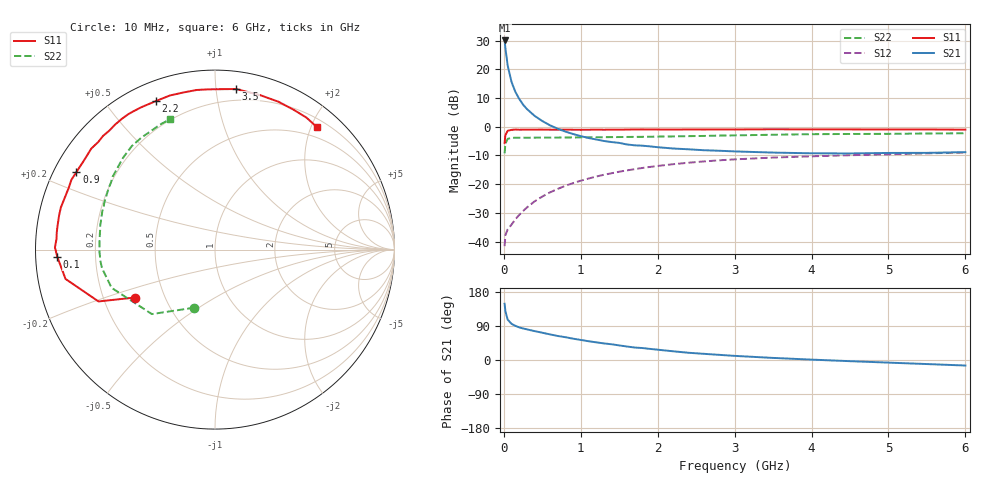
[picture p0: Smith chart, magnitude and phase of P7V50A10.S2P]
! SIEMENS Small Signal Semiconductors
! BFP196
! Si NPN RF Bipolar Junction Transistor in SOT143
! VCE = 0.5 V  IC = 100 mA
! Common Emitter S-Parameters:  May  1996
# GHz  S  MA  R  50
!  f  S11  S21  S12  S22
! GHz  MAG  ANG  MAG  ANG  MAG  ANG  MAG  ANG
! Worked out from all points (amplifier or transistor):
!   36 points, 10 MHz to 6 GHz, reference 50 ohm
!   highest |S21| = 30.0 dB at 10 MHz (marker M1)
!   |S21| within 3 dB of that: start of sweep to 21.79 MHz
!   unconditionally stable (mu >= 1): start of sweep to 16.81 MHz; 119.3 MHz to end of sweep
!   at 250 MHz: K = 1.28, MAG = 15.4 dB, |S12| = -29.4 dB
!   at 1.4 GHz: K = 1.29, MAG = 2.2 dB, |S12| = -16.2 dB
!   at 6 GHz: K = 1.08, MAG = -1.7 dB, |S12| = -9.0 dB
!   S11 on the Smith chart (normalised r, x): 10 MHz: 0.34, -0.25; 100 MHz: 0.06, -0.02; 900 MHz: 0.07, +0.26; 2.2 GHz: 0.08, +0.67; 3.5 GHz: 0.12, +1.13; 6 GHz: 0.33, +2.10
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0.01  0.5217 -149.2  31.75 148.4  0.0083 49.6  0.3433 -109.6
0.02  0.7104 -156.0  23.44 128.9  0.0128 41.2  0.5028 -134.4
0.05  0.8487 -168.9  11.59 106.6  0.0163 35.2  0.6142 -159.7
0.1  0.8797 -177.4  5.998 95.4  0.0197 42.8  0.6379 -170.6
0.15  0.8918 179.2  4.04 90.1  0.0244 49.3  0.6424 -174.7
0.2  0.8851 176.2  3.042 86.1  0.0291 55.0  0.642 -177.0
0.25  0.8868 173.8  2.422 83.2  0.034 58.2  0.6438 -178.8
0.3  0.8872 171.7  2.029 80.9  0.0392 61.0  0.6429 180.0
0.4  0.8893 167.6  1.543 76.2  0.0501 63.1  0.6441 178.0
0.5  0.8903 164.7  1.254 72.0  0.0607 64.3  0.6451 176.3
0.6  0.8854 160.9  1.057 67.6  0.0718 64.4  0.6457 174.8
0.7  0.8847 157.0  0.922 63.4  0.0824 63.7  0.6462 173.4
0.9  0.885 150.8  0.745 56.3  0.1042 61.4  0.6489 170.6
1.1  0.8844 144.1  0.636 49.6  0.1249 58.6  0.6537 168.0
1.6  0.8917 128.6  0.49 35.6  0.1733 49.9  0.6628 161.4
1.8  0.896 122.5  0.467 31.6  0.191 46.0  0.6655 158.6
2.2  0.8906 111.8  0.417 23.0  0.2221 38.9  0.6767 153.0
2.8  0.8952 96.5  0.381 13.6  0.2596 28.6  0.7002 144.5
3.5  0.9024 82.5  0.354 5.5  0.2899 17.5  0.7241 135.0
4.5  0.8964 66.8  0.342 -3.1  0.3186 4.8  0.7466 123.3
5.5  0.8947 55.3  0.35 -10.7  0.3435 -6.0  0.761 113.7
6  0.8876 50.1  0.36 -14.6  0.3545 -11.7  0.7682 109.0
